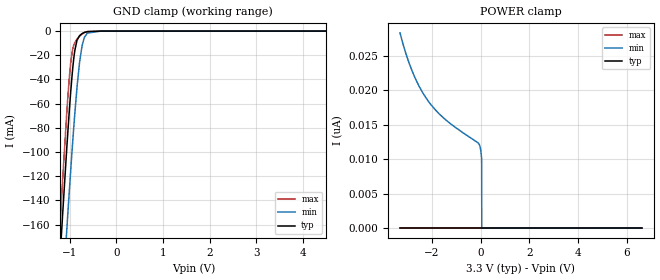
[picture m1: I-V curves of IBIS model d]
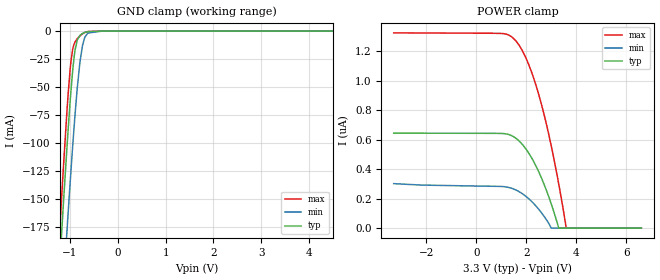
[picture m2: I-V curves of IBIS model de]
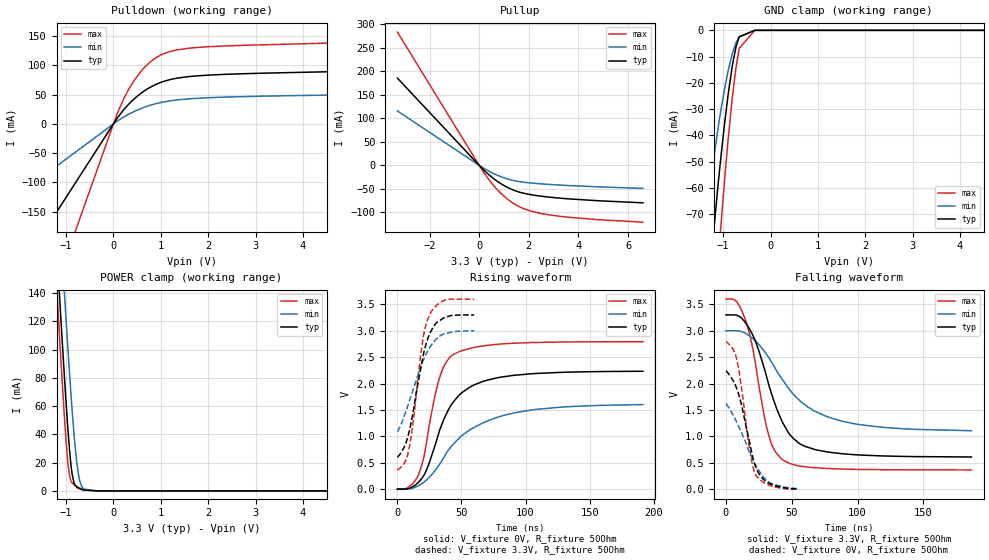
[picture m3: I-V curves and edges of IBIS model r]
|Texas Instruments Incorporated
| SN65HVD7x 3.3-V-Supply Full-Duplex RS-485 with IEC ESD Protection
| Marketing part#   Digital Voltage Range   Package-type   #pins
| SN65HVD70DGS   3.0V-3.6V   VSSOP   10
| SN65HVD70DGSR   3.0V-3.6V   VSSOP   10
| SN65HVD70D   3.0V-3.6V   SOIC   14
| SN65HVD70DR   3.0V-3.6V   SOIC   14
[IBIS Ver]   4.1
[File name]   sn65hvd70.ibs
[File Rev]   1.0
[Date]   6/30/2014
[Source]
| Texas Instruments Incorporated.
| Analog-eLab Design Center, HPA
| 12500 TI Blvd
| Dallas, TX -75243
[Notes]   Revision History:
| Rev 1.0: 6/30/2014
| - Initial version of the model
| - Model generated from simulations in TISPICE
| - Model matched to SPICE simulation
| - C_comp although listed in numerical order of value are
|   obtained from varying PVT conditions. For PVT conditions for
|   each specific value refer the buffer description under
|   respective [Model]. IBIS model user is responsible for using
|   appropriate C_comp to simulate for Signal Integrity.
|* EXCEPTION:   *
|* - For model d, there is leakage current in the GND   *
|*   clamp I-V Table because of the pullup on pad.   *
|* - For model de, there is leakage current in the POWER   *
|*   clamp I-V Table because of the pulldown on pad.   *
|* - For model r, there is leakage current in the POWER   *
|*   clamp I-V Table because of the pulldown on pad.   *
|* - For models a_b_p and a_b_n, there is leakage current in the   *
|*   POWER clamp and GND clamp I-V Table because of the resistor   *
|*   network connected to pad.   *
[Disclaimer]
| This model is designed as an aid for customers of Texas Instruments.
| TI and its licensors and suppliers make no warranties, either expressed
| or implied, with respect to this  model, including the warranties of
| merchantability or fitness for a particular purpose. The model is
| provided solely on an "as is" basis. The entire risk as to its quality
| and performance is with the customer.
[Copyright]
(C) Copyright 2014 Texas Instruments Incorporated.All rights reserved.
|   SN65HVD70DGS
[Component]   SN65HVD70DGS
[Manufacturer]   TI
[Package]   |10 VSSOP  -  DGS package
|   typ   min   max
R_pkg   0.2   0.16   0.24
L_pkg   1.5nH   1.2nH   1.8nH
C_pkg   0.4pF   0.32pF   0.48pF
[Pin]  signal_name   model_name   R_pin   L_pin   C_pin
1   R   r   NA   NA   NA
2   REB   d   NA   NA   NA
3   DE   de   NA   NA   NA
4   D   d   NA   NA   NA
5   GND   gnd   NA   NA   NA
6   Y   y_z_p   NA   NA   NA
7   Z   y_z_n   NA   NA   NA
8   B   a_b_n   NA   NA   NA
9   A   a_b_p   NA   NA   NA
10   VCC   power   NA   NA   NA
[Diff_pin]   inv_pin   vdiff   tdelay_typ   tdelay_min   tdelay_max
6   7   0V   NA   NA   NA
9   8   0.2V   NA   NA   NA
|   SN65HVD70D
[Component]   SN65HVD70D
[Manufacturer]   TI
[Package]   |14 SOIC   -  D package
|   typ   min   max
R_pkg   0.2   0.16   0.24
L_pkg   1.5nH   1.2nH   1.8nH
C_pkg   0.4pF   0.32pF   0.48pF
[Pin]  signal_name   model_name   R_pin   L_pin   C_pin
1   NC   NC   NA   NA   NA
2   R   r   NA   NA   NA
3   REB   d   NA   NA   NA
4   DE   de   NA   NA   NA
5   D   d   NA   NA   NA
6   GND   gnd   NA   NA   NA
7   GND   gnd   NA   NA   NA
8   NC   NC   NA   NA   NA
9   Y   y_z_p   NA   NA   NA
10   Z   y_z_n   NA   NA   NA
11   B   a_b_n   NA   NA   NA
12   A   a_b_p   NA   NA   NA
13   VCC   power   NA   NA   NA
14   VCC   power   NA   NA   NA
[Diff_pin]   inv_pin   vdiff   tdelay_typ   tdelay_min   tdelay_max
9   10   0V   NA   NA   NA
12   11   0.2V   NA   NA   NA
| Models and submodels in the file (7): d (Input), de (Input), r (3-state), a_b_p (Input), a_b_n (Input), y_z_p (Output), y_z_n (Output)
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|   d Model
[Model]   d
Model_type   Input
Vinl = 0.8
Vinh = 2
|   typ   min   max
|   (nom PVT)   (fast PVT)   (slow PVT)
|Average
C_comp   2.275e-12   2.054e-12   2.504e-12
| Where nom  PVT is Nominal Process, 3.3V, 27C
|   Fast PVT is Strong Process,  3.6V, -40C
|   Slow PVT is Weak Process,   3V, 150C
[Voltage Range]   3.3   3   3.6
|Ambient Temperature   25   125   -40
|Junction Temperature
[Temperature Range]   27   150   -40
[Power Clamp Reference]   3.3   3   3.6
[GND Clamp Reference]   0   0   0
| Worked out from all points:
|   GND clamp passes 1 mA (typ) near -0.67 V on its own axis
[GND Clamp]
|   Voltage   I(typ)   I(min)   I(max)
-3.3V     -1.706A    -1.709A    -1.74A
-1.33V    -268.5mA   -332.2mA   -244.5mA
-1.176V   -166.3mA   -233.3mA   -138.2mA
-1.064V   -96.82mA   -164.4mA   -67.68mA
-980.1mV  -50.33mA   -115.2mA   -26.33mA
-945.6mV  -34.42mA   -96.08mA   -16.53mA
-891mV    -15.86mA   -67.76mA   -9.449mA
-789mV    -3.689mA   -25.45mA   -4.166mA
-735mV    -2.045mA   -11.84mA   -2.349mA
-686.4mV  -1.145mA   -5.17mA    -1.213mA
-330mV    -2.214uA   -10.64uA   -3.071uA
6.6V      0A         0A         0A
[POWER Clamp]
|   Voltage   I(typ)   I(min)   I(max)
-3.3V     0A         28.33nA    0A
-3.059V   0A         25.33nA    0A
-2.802V   0A         22.78nA    0A
-2.525V   0A         20.63nA    0A
-2.198V   0A         18.7nA     0A
-1.882V   0A         17.28nA    0A
-1.492V   0A         15.91nA    0A
-42mV     0A         12.06nA    0A
3mV       0A         11.38nA    0A
42mV      0A         10.08nA    0A
51mV      0A         0A         0A
6.6V      0A         0A         0A
|   de Model
[Model]   de
Model_type   Input
Vinl = 0.8
Vinh = 2.0
|   typ   min   max
|   (nom PVT)   (fast PVT)   (slow PVT)
|Average
C_comp   2.269e-12   2.052e-12   2.501e-12
| Where nom  PVT is Nominal Process, 3.3V, 27C
|   Fast PVT is Strong Process,  3.6V, -40C
|   Slow PVT is Weak Process,   3V, 150C
[Voltage Range]   3.3   3   3.6
|Ambient Temperature   25   125   -40
|Junction Temperature
[Temperature Range]   27   150   -40
[Power Clamp Reference]   3.3   3   3.6
[GND Clamp Reference]   0   0   0
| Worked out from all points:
|   GND clamp passes 1 mA (typ) near -0.67 V on its own axis
[GND Clamp]
|   Voltage   I(typ)   I(min)   I(max)
-3.3V     -1.874A    -1.882A    -1.904A
-1.324V   -288.6mA   -359.8mA   -260.8mA
-1.176V   -180.8mA   -255.1mA   -149.1mA
-1.065V   -104.7mA   -179.5mA   -72.15mA
-980.1mV  -53.39mA   -124.8mA   -26.97mA
-945.6mV  -36.1mA    -103.7mA   -16.67mA
-891mV    -16.24mA   -72.63mA   -9.451mA
-792mV    -3.818mA   -27.65mA   -4.283mA
-693mV    -1.245mA   -5.894mA   -1.338mA
-627mV    -485.8uA   -1.777mA   -431.7uA
-330mV    -858.8nA   -10.04uA   -475.9nA
6.6V      0A         0A         0A
[POWER Clamp]
|   Voltage   I(typ)   I(min)   I(max)
-3.3V     644.8nA    302.2nA    1.325uA
933.9mV   643nA      283.5nA    1.322uA
1.412V    628nA      270.8nA    1.299uA
1.729V    588.8nA    246.1nA    1.237uA
1.971V    540.7nA    217.8nA    1.16uA
2.241V    468.8nA    176.7nA    1.045uA
2.507V    379nA      126nA      901.4nA
2.76V     276.3nA    68.43nA    737nA
2.996V    165nA      0A         559.3nA
3.297V    0A         0A         300.1nA
3.598V    0A         0A         0A
6.6V      0A         0A         0A
|   r Model
[Model]   r
Model_type   3-state
Polarity   Non-Inverting
Vmeas = 1.65
Vref = 0
Cref = 2pF
Rref = 70
|   typ   min   max
|   (nom PVT)   (fast PVT)   (slow PVT)
C_comp   2.259e-12   1.803e-12   2.415e-12
| Where nom  PVT is Nominal Process, 3.3V, 27C
|   Fast PVT is Strong Process,  3.6V, -40C
|   Slow PVT is Weak Process,   3V, 150C
[Voltage Range]   3.3   3   3.6
|Ambient Temperature   25   125   -40
|Junction Temperature
[Temperature Range]   27   150   -40
[Pullup Reference]   3.3   3   3.6
[Pulldown Reference]   0   0   0
[Power Clamp Reference]   3.3   3   3.6
[GND Clamp Reference]   0   0   0
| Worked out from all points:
|   slope of the pulldown table from 0 to 0.495 V, typ, clamps not added: 10.6 ohm
|   slope of the pullup table from 0 to 0.495 V, typ, clamps not added: 20.2 ohm
|   POWER clamp passes 1 mA (typ) near -0.67 V on its own axis
|   falling waveform, V_fixture 3.3V, R_fixture 50Ohm: 20-80 % time 22.7ns typ, 38.2ns min, 14.9ns max; typ from 3.3 V to 0.609 V
|   rising waveform, V_fixture 0V, R_fixture 50Ohm: 20-80 % time 24.4ns typ, 41ns min, 14.6ns max; typ from 0 V to 2.23 V
|   rising waveform, V_fixture 3.3V, R_fixture 50Ohm: 20-80 % time 12.8ns typ, 17ns min, 9.87ns max; typ from 0.607 V to 3.3 V
|   falling waveform, V_fixture 0V, R_fixture 50Ohm: 20-80 % time 12.5ns typ, 18ns min, 9.46ns max; typ from 2.24 V to 0.002 V
[Pulldown]
|   Voltage   I(typ)   I(min)   I(max)
-3.3V     -414.6mA   -198.7mA   -753.2mA
-2.4mV    -301.5uA   -144.5uA   -547.8uA
206.4mV   23.02mA    11.26mA    40.8mA
462mV     44.53mA    22.24mA    77.04mA
746.4mV   61.21mA    31.15mA    103.6mA
1.046V    72.25mA    37.37mA    119.5mA
1.353V    78.31mA    41.11mA    126.6mA
1.821V    82.45mA    44.04mA    130.9mA
4.912V    89.8mA     49.78mA    138.9mA
5.581V    92.27mA    51.1mA     143.1mA
6.136V    97.15mA    53.46mA    151.8mA
6.6V      105.2mA    57.34mA    166mA
[GND Clamp]
|   Voltage   I(typ)   I(min)   I(max)
-3.3V     -1.049A    -411mA     -1.939A
-1.435V   -125mA     -81.46mA   -173.6mA
-1.298V   -95.82mA   -61.81mA   -136.1mA
-1.097V   -57.08mA   -36.08mA   -86.15mA
-1.035V   -46.31mA   -29.12mA   -71.81mA
-966mV    -35.09mA   -21.99mA   -56.51mA
-894.3mV  -24.52mA   -15.43mA   -41.68mA
-810mV    -13.95mA   -9.11mA    -26.27mA
-729.3mV  -6.389mA   -4.763mA   -14.35mA
-661.2mV  -2.512mA   -2.447mA   -6.887mA
-330mV    -901.7nA   -10.64uA   -1.037uA
6.6V      0A         0A         0A
[Pullup]
|   Voltage   I(typ)   I(min)   I(max)
-3.3V     185.9mA    115.9mA    283.8mA
159.6mV   -8.64mA    -5.383mA   -13.18mA
656.7mV   -31.16mA   -19.34mA   -47.56mA
1.128V    -46.6mA    -28.71mA   -71.43mA
1.445V    -53.9mA    -32.95mA   -83.1mA
1.731V    -58.52mA   -35.47mA   -90.8mA
2.183V    -63.24mA   -37.98mA   -98.74mA
2.721V    -67.04mA   -40.18mA   -104.6mA
3.633V    -71.43mA   -43.01mA   -110.6mA
6.6V      -79.71mA   -48.99mA   -121mA
[POWER Clamp]
|   Voltage   I(typ)   I(min)   I(max)
-3.3V     1.523A     1.552A     1.524A
-1.277V   221.3mA    279.6mA    193.7mA
-1.136V   138mA      197.7mA    109mA
-1.033V   80.29mA    139.6mA    51.63mA
-950.4mV  39.51mA    95.71mA    16.73mA
-871.2mV  11.99mA    57.3mA     5.692mA
-831mV    5.651mA    40.15mA    4.418mA
-771mV    2.525mA    19.5mA     3.125mA
-722.7mV  1.633mA    8.844mA    2.248mA
-621mV    581.5uA    1.307mA    824.5uA
-330mV    1.405uA    13.07uA    470.9nA
6.6V      0A         0A         0A
[Ramp]
R_load = 50
|   typ   min   max
dV/dt_r   1.34292/2.44848e-08   0.968415/4.16883e-08   1.6774/1.45071e-08
dV/dt_f   1.61594/2.25532e-08   1.14324/3.86691e-08   1.94165/1.48447e-08
[Falling Waveform]
V_fixture = 3.3V
V_fixture_min = 3V
V_fixture_max = 3.6V
R_fixture = 50Ohm
|   Time   V(typ)   V(min)   V(max)
0s        3.3V       3V         3.6V
8.2ns     3.293V     2.999V     3.548V
15.85ns   3.117V     2.939V     3.132V
22.75ns   2.78V      2.799V     2.332V
29.2ns    2.282V     2.612V     1.374V
32.5ns    1.984V     2.494V     1.025V
42.9ns    1.27V      2.075V     558.9mV
56.7ns    851mV      1.663V     435mV
87.95ns   671.7mV    1.289V     380.8mV
186.6ns   609.1mV    1.106V     364.2mV
[Rising Waveform]
V_fixture = 0V
V_fixture_min = 0V
V_fixture_max = 0V
R_fixture = 50Ohm
|   Time   V(typ)   V(min)   V(max)
0s        1.908nV    301.7nV    275.6pV
9.5ns     16.7mV     4.776mV    49.62mV
16.45ns   130mV      63.38mV    268.9mV
20.7ns    259.8mV    132.6mV    615.7mV
31.6ns    1.003V     424.3mV    1.999V
36.5ns    1.334V     609.3mV    2.339V
42.8ns    1.623V     828.4mV    2.538V
59.55ns   1.972V     1.165V     2.684V
90.8ns    2.157V     1.444V     2.765V
191.5ns   2.235V     1.603V     2.795V
[Rising Waveform]
V_fixture = 3.3V
V_fixture_min = 3V
V_fixture_max = 3.6V
R_fixture = 50Ohm
|   Time   V(typ)   V(min)   V(max)
0s        606.8mV    1.095V     363.9mV
5.7ns     819.4mV    1.41V      505.2mV
9.25ns    1.097V     1.661V     782.6mV
12.5ns    1.49V      1.9V       1.306V
15.9ns    1.979V     2.151V     2.094V
20.3ns    2.546V     2.449V     2.899V
23.95ns   2.867V     2.632V     3.237V
29.15ns   3.113V     2.813V     3.445V
36.2ns    3.245V     2.94V      3.573V
59.95ns   3.3V       3.002V     3.6V
[Falling Waveform]
V_fixture = 0V
V_fixture_min = 0V
V_fixture_max = 0V
R_fixture = 50Ohm
|   Time   V(typ)   V(min)   V(max)
0s        2.238V     1.614V     2.796V
5.3ns     2.063V     1.408V     2.655V
8.6ns     1.878V     1.245V     2.417V
12.25ns   1.552V     1.047V     1.849V
17.1ns    985.4mV    751.2mV    897.4mV
20.45ns   597.8mV    558mV      429.9mV
22.4ns    438.8mV    464.7mV    284.6mV
25.55ns   275.2mV    332.5mV    193.6mV
30.85ns   133mV      168.9mV    97.35mV
55.2ns    1.654mV    7.294mV    -364uV
